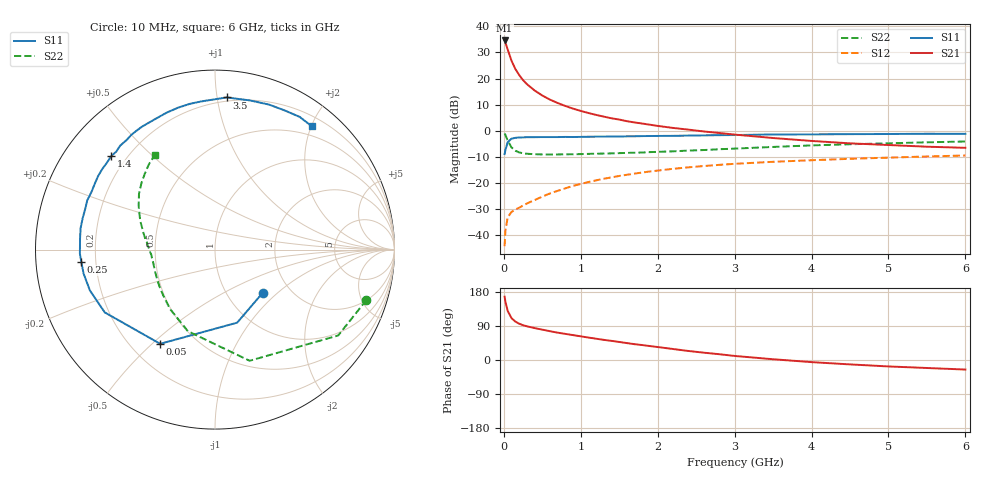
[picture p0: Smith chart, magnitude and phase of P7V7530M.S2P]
! SIEMENS Small Signal Semiconductors
! BFP196
! Si NPN RF Bipolar Junction Transistor in SOT143
! VCE = 0.75 V  IC = 30 mA
! Common Emitter S-Parameters:  May  1996
# GHz  S  MA  R  50
!  f  S11  S21  S12  S22
! GHz  MAG  ANG  MAG  ANG  MAG  ANG  MAG  ANG
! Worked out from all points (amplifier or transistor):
!   36 points, 10 MHz to 6 GHz, reference 50 ohm
!   highest |S21| = 34.6 dB at 10 MHz (marker M1)
!   |S21| within 3 dB of that: start of sweep to 44.91 MHz
!   unconditionally stable (mu >= 1): 489 MHz to end of sweep
!   at 250 MHz: K = 0.76, MSG = 24.0 dB, |S12| = -28.6 dB
!   at 1.4 GHz: K = 1.11, MAG = 9.2 dB, |S12| = -17.8 dB
!   at 6 GHz: K = 1.03, MAG = 0.4 dB, |S12| = -9.5 dB
!   S11 on the Smith chart (normalised r, x): 10 MHz: 1.46, -0.81; 50 MHz: 0.32, -0.53; 250 MHz: 0.14, -0.04; 1.4 GHz: 0.14, +0.38; 3.5 GHz: 0.17, +1.06; 6 GHz: 0.35, +2.00
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0.01  0.3586 -42.3  53.46 167.2  0.0062 77.5  0.8895 -18.4
0.02  0.4254 -73.1  49.11 154.4  0.0121 66.2  0.8365 -34.9
0.05  0.6073 -120.2  35.89 129.6  0.0221 49.6  0.6487 -72.7
0.1  0.7068 -150.3  21.79 110.4  0.028 39.6  0.479 -108.4
0.15  0.7332 -161.9  15.2 101.4  0.0312 38.8  0.4152 -127.0
0.2  0.7444 -169.7  11.62 95.7  0.0338 41.7  0.3853 -138.5
0.25  0.7479 -174.8  9.298 91.8  0.0371 44.0  0.3709 -146.8
0.3  0.7531 -178.3  7.8 88.9  0.0406 47.0  0.3635 -151.9
0.4  0.7545 175.2  5.897 84.2  0.0473 50.7  0.3559 -159.5
0.5  0.7583 170.9  4.726 80.1  0.055 53.4  0.3528 -164.3
0.6  0.7578 166.4  3.944 76.0  0.0633 54.8  0.3519 -167.7
0.7  0.7579 162.2  3.396 72.1  0.071 55.4  0.3528 -170.4
0.9  0.7595 155.1  2.652 65.7  0.0884 55.6  0.3552 -174.6
1.1  0.7692 148.0  2.186 59.2  0.1045 54.9  0.3616 -177.6
1.4  0.7781 138.0  1.733 50.5  0.1285 51.8  0.3697 178.4
1.7  0.7845 128.8  1.444 41.7  0.1517 48.1  0.3806 174.3
2.2  0.7994 115.2  1.134 29.0  0.1871 41.2  0.4045 168.1
3  0.829 95.4  0.846 10.7  0.2334 29.5  0.4557 156.8
3.5  0.8502 85.6  0.727 2.0  0.255 22.8  0.4908 150.1
4.5  0.8622 69.6  0.575 -11.6  0.2908 10.9  0.5524 137.9
5.5  0.8771 57.4  0.496 -21.1  0.3223 0.2  0.6017 127.7
6  0.8734 52.0  0.472 -25.2  0.3366 -5.6  0.6238 122.5
